(* Logix 5000 Rung export; software revision 24.00 *)

TYPE SNAPP_CONTROL_22 :
STRUCT
   Reserved_0_0 : BOOL;
   Trigger : BOOL;
   Reserved_0_2 : BOOL;
   InspectionResultsAck : BOOL;
   ExecuteCommand : BOOL;
   Reserved_0_5 : BOOL;
   Reserved_0_6 : BOOL;
   Reserved_0_7 : BOOL;
   Reserved_Byte1 : SINT;
   Reserved_2_0 : BOOL;
   Reserved_2_1 : BOOL;
   ClearError : BOOL;
   Reserved_2_3 : BOOL;
   Reserved_2_4 : BOOL;
   Reserved_2_5 : BOOL;
   Reserved_2_6 : BOOL;
   Reserved_2_7 : BOOL;
   Reserved_3_0 : BOOL;
   Reserved_3_1 : BOOL;
   Reserved_3_2 : BOOL;
   Reserved_3_3 : BOOL;
   Reserved_3_4 : BOOL;
   Reserved_3_5 : BOOL;
   Reserved_3_6 : BOOL;
   Reserved_3_7 : BOOL;
   CommandID : INT;
   Reserved_Bytes6and7 : INT;
END_STRUCT
END_TYPE

TYPE SNAPP_IN_13 :
STRUCT
   Status : SNAPP_STAT_IN_13;
   InspectionResults : SNAPP_RESULTS_13;
END_STRUCT
END_TYPE

TYPE SNAPP_STAT_IN_13 :
STRUCT
   TriggerReady : BOOL;
   TriggerAck : BOOL;
   Reserved_0_2 : BOOL;
   AcqError : BOOL;
   Reserved_0_4 : BOOL;
   Reserved_0_5 : BOOL;
   Reserved_0_6 : BOOL;
   Online : BOOL;
   Reserved_1_0 : BOOL;
   InspectionCompleted : BOOL;
   Reserved_1_2 : BOOL;
   ResultsValid : BOOL;
   CommandExecuting : BOOL;
   CommandCompleted : BOOL;
   CommandFailed : BOOL;
   Error : BOOL;
   Reserved_2_0 : BOOL;
   Reserved_2_1 : BOOL;
   Reserved_2_2 : BOOL;
   Reserved_2_3 : BOOL;
   InspectionPass : BOOL;
   Reserved_2_5 : BOOL;
   Reserved_2_6 : BOOL;
   Reserved_2_7 : BOOL;
   Reserved_3_0 : BOOL;
   Reserved_3_1 : BOOL;
   Reserved_3_2 : BOOL;
   Reserved_3_3 : BOOL;
   Reserved_3_4 : BOOL;
   Reserved_3_5 : BOOL;
   Reserved_3_6 : BOOL;
   Reserved_3_7 : BOOL;
   ErrorID : INT;
   Reserved_Bytes_6_7 : INT;
   CurrentProgramID : INT;
   AcquisitionID : INT;
   InspectionID : INT;
   Reserved_Bytes_14_15 : INT;
END_STRUCT
END_TYPE

TYPE SNAPP_RESULTS_13 :   // Inspection Results from Sensor
STRUCT
   PayloadVersion : SINT;
   ApplicationType : SINT;   // 0=Error, 1=Anomaly Detection, 2=Binary Classifier, 3=4-Class Binary Classifier, 4...255=Reserved
   Program : SINT;
   InspectionStatusCode : SINT;   // 0=Inspection Valid, 1=Sensor Untrained, 2=Fixture Not Found, 3=ROI Outside Image, 4...255=Reserved
   IdentifiedClassEnum : SINT;   // Anomaly: 0=Reserved, 1=OK, 2=NG, 3-254=Reserved, 255=Error
   IdentifiedClassConfidence : SINT;
   ClassName : SINT[474];
END_STRUCT
END_TYPE

TYPE SNAPP_OUT_22 :
STRUCT
   Control : SNAPP_CONTROL_22;
END_STRUCT
END_TYPE

TYPE SNAPP_PartResults :
STRUCT
   InspectionPass : BOOL;
   InspectionID : INT;
   Result : SNAPP_RESULTS_13;
END_STRUCT
END_TYPE

VAR_GLOBAL   (* controller tags *)
   Part_Results : SNAPP_PartResults;
   SNAPP2800_Out : SNAPP_OUT_22 := (Control.CommandID := 1);
   sbRV : BOOL;
   SNAPP2800_In : SNAPP_IN_13;
END_VAR

PROGRAM MainProgram

ROUTINE SNAPPky   (* ladder *)
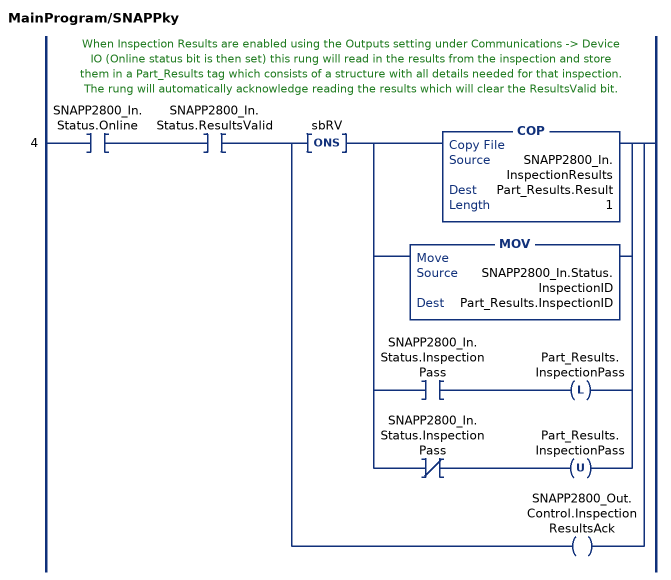
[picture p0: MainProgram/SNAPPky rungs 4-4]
   // When Inspection Results are enabled using the Outputs setting under Communications -> Device IO (Online status bit is then set) this rung will read in the results from the inspection and store them in a Part_Results tag which consists of a structure with all details needed for that inspection.   The rung will automatically acknowledge reading the results which will clear the ResultsValid bit.
   4: XIC(SNAPP2800_In.Status.Online)XIC(SNAPP2800_In.Status.ResultsValid)[ONS(sbRV) [COP(SNAPP2800_In.InspectionResults,Part_Results.Result,1) ,MOV(SNAPP2800_In.Status.InspectionID,Part_Results.InspectionID) ,XIC(SNAPP2800_In.Status.InspectionPass) OTL(Part_Results.InspectionPass) ,XIO(SNAPP2800_In.Status.InspectionPass) OTU(Part_Results.InspectionPass) ] ,OTE(SNAPP2800_Out.Control.InspectionResultsAck) ];
END_ROUTINE
END_PROGRAM
